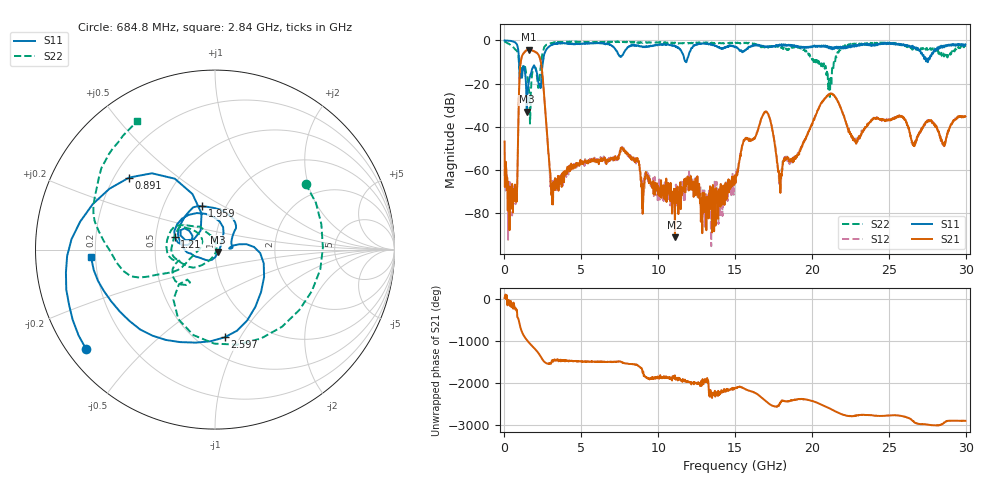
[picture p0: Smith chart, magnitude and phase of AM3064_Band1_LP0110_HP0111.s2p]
# Hz S DB R 50.0
!freq dBS11 angS11 dBS21 angS21 dBS12 angS12 dBS22 angS22
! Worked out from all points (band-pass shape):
!   1600 points, 10 MHz to 29.98 GHz, reference 50 ohm
!   highest |S21| = -4.26 dB at 1.584 GHz (marker M1); lowest = -91.2 dB at 11.09 GHz (marker M2)
!   |S21| within 3 dB of the highest: 1.142 GHz to 2.257 GHz (1.114 GHz wide, 65.6 % of centre)
!   lowest |S11| = -33.0 dB at 1.453 GHz (marker M3), VSWR 1.05, Z = 51.8 - j1.36 ohm
!   |S11| at or under -10 dB: 949.5 MHz to 2.504 GHz (1.555 GHz wide, 90 % of centre); 11.80844 GHz to 11.83234 GHz (23.91 MHz wide, 0.202 % of centre); 27.53235 GHz to 27.54629 GHz (13.94 MHz wide, 0.0506 % of centre)
!   |S22| runs from -38.5 to -0.4 dB; largest |S21 - S12| = 0.0087
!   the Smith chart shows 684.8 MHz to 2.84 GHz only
!   S11 on the Smith chart (normalised r, x): 684.8 MHz: 0.05, -0.34; 891 MHz: 0.26, +0.34; 1.21 GHz: 0.63, +0.09; 1.959 GHz: 0.78, +0.40; 2.597 GHz: 0.67, -0.86; 2.84 GHz: 0.18, -0.03
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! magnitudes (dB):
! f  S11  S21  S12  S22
! 10 MHz  0.0  -46.8  -59.6  -0.4
! 684.8 MHz  -0.8  -66.7  -74.4  -4.1
! 891 MHz  -4.1  -42.7  -42.0  -6.2
! 1.21 GHz  -12.6  -6.3  -6.2  -11.8
! 1.453 GHz  -33.0  -4.5  -4.5  -16.2
! 1.584 GHz  -19.0  -4.3  -4.2  -21.9
! 1.959 GHz  -12.0  -5.1  -5.1  -12.5
! 2.597 GHz  -6.2  -27.0  -27.0  -3.0
! 2.84 GHz  -3.2  -49.7  -49.8  -1.6
! 3.178 GHz  -1.8  -65.7  -66.9  -1.0
! 5.015 GHz  -1.5  -56.2  -56.3  -0.7
! 7.714 GHz  -6.5  -50.1  -50.2  -0.8
! 10 GHz  -2.0  -67.4  -67.9  -1.0
! 11.09 GHz  -2.6  -91.2  -74.6  -1.0
! 15 GHz  -3.1  -64.4  -65.8  -1.4
! 16.94 GHz  -2.8  -33.4  -33.1  -3.2
! 17.93 GHz  -2.1  -65.7  -65.8  -2.7
! 19.99 GHz  -3.2  -38.8  -39.0  -8.4
! 21.21 GHz  -3.8  -24.7  -24.6  -17.4
! 22.8 GHz  -2.2  -46.5  -45.8  -2.0
! 25 GHz  -1.1  -36.9  -36.5  -1.3
! 29.98 GHz  -1.9  -35.3  -35.6  -2.9
